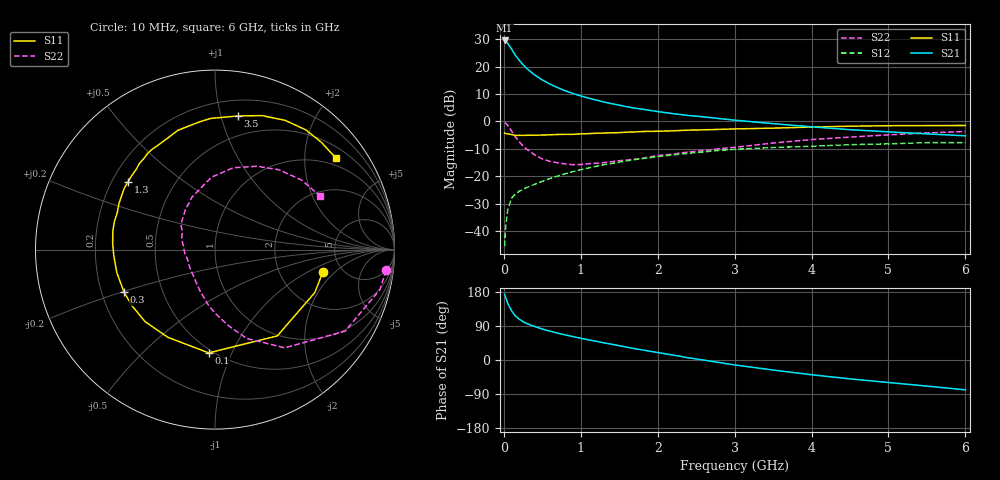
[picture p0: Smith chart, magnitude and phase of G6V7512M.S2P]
! SIEMENS Small Signal Semiconductors
! BFG193
! Si NPN RF Bipolar Junction Transistor in SOT223
! VCE = 0.75 V  IC = 12 mA
! Common Emitter S-Parameters:  August  1996
# GHz  S  MA  R  50
!  f  S11  S21  S12  S22
! GHz  MAG  ANG  MAG  ANG  MAG  ANG  MAG  ANG
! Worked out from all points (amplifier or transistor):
!   36 points, 10 MHz to 6 GHz, reference 50 ohm
!   highest |S21| = 29.6 dB at 10 MHz (marker M1)
!   |S21| within 3 dB of that: start of sweep to 96.74 MHz
!   unconditionally stable (mu >= 1): 757.6 MHz to 3.91 GHz
!   at 250 MHz: K = 0.61, MSG = 22.7 dB, |S12| = -24.8 dB
!   at 1.4 GHz: K = 1.08, MAG = 9.2 dB, |S12| = -15.3 dB
!   at 6 GHz: K = 0.98, MSG = 1.2 dB, |S12| = -7.7 dB
!   S11 on the Smith chart (normalised r, x): 10 MHz: 3.58, -1.42; 100 MHz: 0.48, -0.82; 300 MHz: 0.30, -0.20; 1.3 GHz: 0.27, +0.32; 3.5 GHz: 0.33, +1.13; 6 GHz: 0.78, +2.77
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0.01  0.6141 -11.6  30.09 173.3  0.0053 85.6  0.9603 -6.9
0.02  0.6055 -23.3  29.68 167.6  0.0104 79.6  0.9452 -13.7
0.05  0.593 -54.2  26.76 149.6  0.0242 67.6  0.8554 -32.1
0.1  0.5764 -93.5  20.97 130.1  0.0396 55.3  0.6716 -54.6
0.15  0.5549 -118.4  16.15 116.1  0.0474 48.1  0.5259 -70.3
0.2  0.5592 -134.3  13.07 107.8  0.0532 46.2  0.4279 -80.3
0.25  0.5581 -145.9  10.81 101.1  0.0578 45.2  0.3553 -89.8
0.3  0.5595 -154.8  9.21 96.1  0.0625 45.4  0.3101 -97.0
0.4  0.5619 -166.9  7.071 88.5  0.0713 46.4  0.2455 -109.8
0.5  0.5649 -176.6  5.707 81.7  0.0808 46.8  0.2072 -121.1
0.6  0.5711 176.6  4.801 76.1  0.0908 47.5  0.187 -131.0
0.7  0.5784 169.9  4.139 70.8  0.1008 47.4  0.1762 -140.7
0.8  0.582 164.7  3.62 66.2  0.1111 46.6  0.1679 -150.3
1.1  0.6001 150.3  2.667 53.3  0.1416 44.1  0.1694 -172.8
1.3  0.6143 142.3  2.269 45.3  0.1623 41.2  0.1767 173.4
1.7  0.6436 128.1  1.751 29.9  0.2008 34.0  0.2048 153.2
2.2  0.6753 112.8  1.388 13.0  0.2463 23.1  0.2537 134.7
2.8  0.7176 96.6  1.13 -6.7  0.2963 9.8  0.3186 113.9
3.5  0.7558 80.2  0.913 -26.5  0.3347 -7.3  0.4041 92.8
4.5  0.8194 61.5  0.708 -49.8  0.3773 -26.2  0.519 63.5
5.5  0.8416 45.3  0.594 -68.9  0.4108 -48.3  0.6187 38.8
6  0.8447 37.3  0.547 -78.7  0.4107 -60.8  0.6572 27.0
